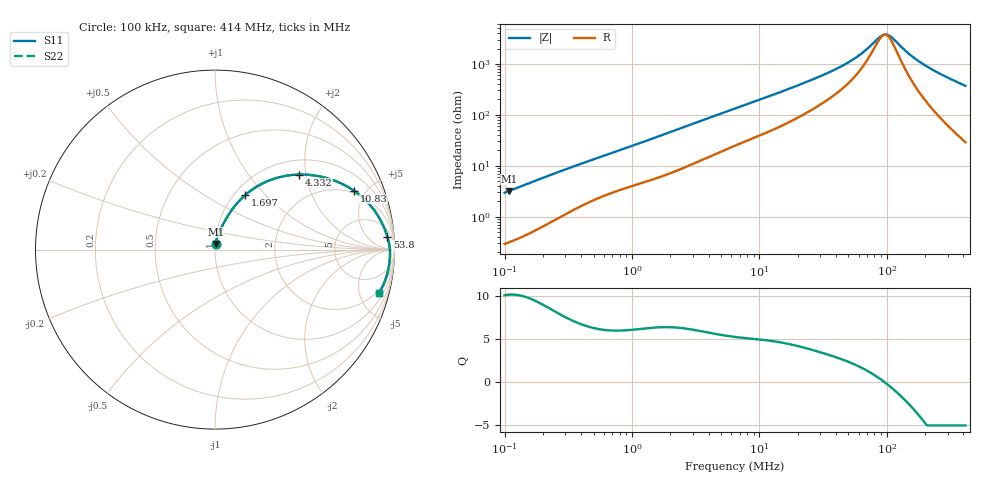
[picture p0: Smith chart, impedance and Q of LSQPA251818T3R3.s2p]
! LSQPA251818T3R3  S-PARAMETER MODEL  ( General Type )
! Model Generated by TAIYO YUDEN Corporation (http://www.ty-top.com)
! Version 3.0
! TAIYO YUDEN Control No. 160907NF25SB-FKC
! Copyright(c) 2007 TAIYO YUDEN CO.,LTD. All Rights Reserved.
! Product Description (link to TY-COMPAS)
! https://ds.yuden.co.jp/TYCOMPAS/or/detail?pn=LSQPA251818T3R3M&u=M
! Products Name : Inductors
! Characteristics :
!  Inductance : 3.3 uH , SRF(min) : 54 MHz , DC Resistance(max) : 0.208 Ohm
!  Rated Current : Saturation :730 mA , Temp Rise : 1020 mA (40 degC)
!  Case Size : 2.5 x 1.8 / 0.098 x 0.071 [mm/inch] , Thickness : 1.8 / 0.071 [mm/inch]
!  (Conditions: Temperature = 25 degC , DC Bias Current/Voltage = 0A / 0V)
! External Node Assignments :
!  1  o---GGG---o  2
! GND o---------o GND
! Frequency Range : 0.1MHz  -  413.982163MHz  [ 402 STEP ]
# MHz S RI R 50
! Freq[MHz].  S11 Real  S11 Imag  S21 Real  S21 Imag  S12 Real  S12 Imag  S22 Real  S22 Imag
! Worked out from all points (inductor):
!   401 points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, 100 kHz to 414 MHz, reference 50 ohm
!   read as one part in series: L = 4.64 uH near 104.3 kHz
!   highest Q = 10.1 at 108.7 kHz (marker M1), where L = 4.66 uH
!   self-resonance near 96.29 MHz
!   S11 on the Smith chart (normalised r, x): 100 kHz: 1.01, +0.06; 1.697 MHz: 1.12, +0.78; 4.332 MHz: 1.32, +1.83; 10.83 MHz: 1.85, +4.14; 53.8 MHz: 11, +22; 414 MHz: 1.58, -7.39
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0.1  0.00375 0.0291  0.9962 -0.0291  0.9962 -0.0291  0.00375 0.0291
0.108685  0.00413 0.0316  0.9959 -0.0316  0.9959 -0.0316  0.00413 0.0316
0.403501  0.0274 0.1047  0.9726 -0.1047  0.9726 -0.1047  0.0274 0.1047
0.908867  0.0777 0.1972  0.9223 -0.1972  0.9223 -0.1972  0.0777 0.1972
1.628129  0.161 0.2972  0.839 -0.2972  0.839 -0.2972  0.161 0.2972
1.697359  0.1697 0.3049  0.8303 -0.3049  0.8303 -0.3049  0.1697 0.3049
2.856506  0.3155 0.3903  0.6845 -0.3903  0.6845 -0.3903  0.3155 0.3903
4.331958  0.4687 0.4182  0.5313 -0.4182  0.5313 -0.4182  0.4687 0.4182
6.434145  0.6151 0.4005  0.3849 -0.4005  0.3849 -0.4005  0.6151 0.4005
10.8281  0.7743 0.3281  0.2257 -0.3281  0.2257 -0.3281  0.7743 0.3281
16.42106  0.861 0.2518  0.139 -0.2518  0.139 -0.2518  0.861 0.2518
25.96183  0.9178 0.1718  0.0822 -0.1718  0.0822 -0.1718  0.9178 0.1718
39.37171  0.9472 0.1106  0.0528 -0.1106  0.0528 -0.1106  0.9472 0.1106
53.80481  0.9611 0.0704  0.0389 -0.0704  0.0389 -0.0704  0.9611 0.0704
66.25912  0.9675 0.045  0.0325 -0.045  0.0325 -0.045  0.9675 0.045
90.54875  0.9735 0.00747  0.0265 -0.00747  0.0265 -0.00747  0.9735 0.00747
98.41296  0.9744 -0.00266  0.0256 0.00266  0.0256 0.00266  0.9744 -0.00266
104.7562  0.9748 -0.0103  0.0252 0.0103  0.0252 0.0103  0.9748 -0.0103
149.2455  0.974 -0.0563  0.026 0.0563  0.026 0.0563  0.974 -0.0563
187.6586  0.9699 -0.0894  0.0301 0.0894  0.0301 0.0894  0.9699 -0.0894
272.9811  0.9545 -0.153  0.0455 0.153  0.0455 0.153  0.9545 -0.153
413.9822  0.9158 -0.2413  0.0842 0.2413  0.0842 0.2413  0.9158 -0.2413
